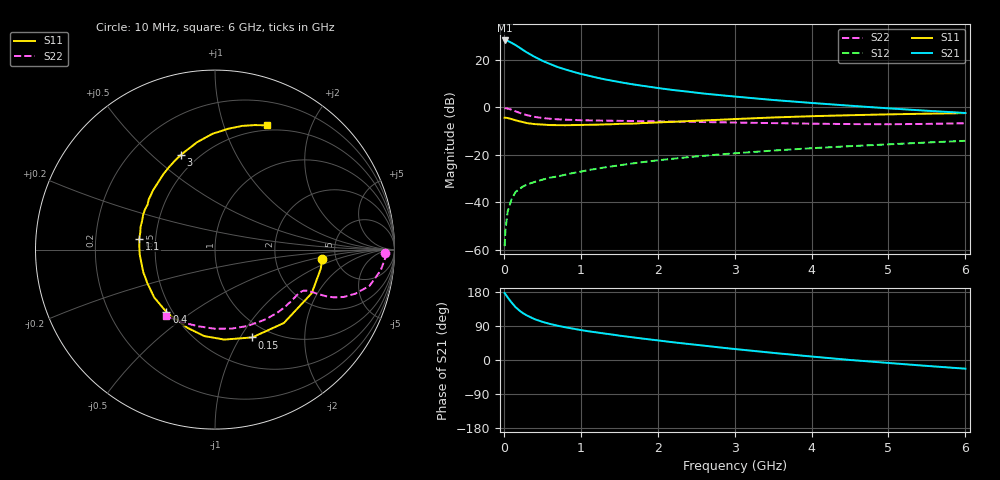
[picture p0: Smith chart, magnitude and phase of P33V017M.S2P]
! SIEMENS Small Signal Semiconductors
! BFP181
! Si NPN RF Bipolar Junction Transistor in SOT143
! VCE = 3 V  IC = 17 mA
! Common Emitter S-Parameters:  March  1996
# GHz  S  MA  R  50
!  f  S11  S21  S12  S22
! GHz  MAG  ANG  MAG  ANG  MAG  ANG  MAG  ANG
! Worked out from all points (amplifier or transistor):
!   36 points, 10 MHz to 6 GHz, reference 50 ohm
!   highest |S21| = 28.0 dB at 10 MHz (marker M1)
!   |S21| within 3 dB of that: start of sweep to 203.9 MHz
!   unconditionally stable (mu >= 1): start of sweep to 11.11 MHz; 618.9 MHz to end of sweep
!   at 250 MHz: K = 0.55, MSG = 28.7 dB, |S12| = -33.4 dB
!   at 1.4 GHz: K = 1.32, MAG = 14.7 dB, |S12| = -24.9 dB
!   at 6 GHz: K = 1.07, MAG = 4.3 dB, |S12| = -14.2 dB
!   S11 on the Smith chart (normalised r, x): 10 MHz: 3.88, -0.62; 150 MHz: 0.83, -1.13; 400 MHz: 0.46, -0.40; 1.1 GHz: 0.40, +0.06; 3 GHz: 0.40, +0.63; 6 GHz: 0.44, +1.40
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0.01  0.5987 -4.9  25.19 176.8  0.0012 83.5  0.9487 -1.1
0.02  0.599 -10.2  25.14 174.1  0.0025 80.1  0.9503 -2.7
0.05  0.5911 -24.3  24.63 165.1  0.0065 83.3  0.9308 -7.1
0.1  0.5608 -46.8  22.5 151.7  0.0116 68.2  0.8843 -13.2
0.15  0.5315 -67.0  20.27 140.0  0.0163 63.6  0.8203 -17.4
0.2  0.504 -84.1  18.01 130.8  0.0191 58.5  0.7643 -20.2
0.25  0.4853 -97.2  15.86 123.4  0.0215 55.3  0.7168 -21.8
0.3  0.4619 -109.6  14.1 117.5  0.0237 54.5  0.6789 -22.7
0.4  0.4406 -127.9  11.4 107.8  0.0269 52.5  0.6254 -23.3
0.5  0.431 -141.8  9.434 100.8  0.0299 51.3  0.5917 -23.6
0.6  0.4207 -153.3  8.077 95.2  0.033 51.9  0.5704 -23.9
0.7  0.4188 -162.4  6.952 90.4  0.0351 52.7  0.5552 -24.3
0.9  0.4203 -176.4  5.547 82.7  0.0413 53.9  0.5382 -25.5
1.1  0.426 171.7  4.583 75.8  0.0478 54.4  0.5272 -27.4
1.5  0.445 154.1  3.369 64.4  0.0601 54.9  0.5154 -32.1
1.8  0.4633 142.9  2.816 56.6  0.0698 54.4  0.5076 -36.4
2.2  0.4916 129.9  2.292 46.8  0.0825 52.3  0.4982 -42.6
3  0.5619 109.6  1.67 29.0  0.1073 47.2  0.4744 -56.9
3.5  0.6069 99.4  1.415 18.8  0.1224 43.8  0.4623 -67.0
4.5  0.6768 83.9  1.072 0.1  0.1514 35.7  0.4411 -90.1
5.5  0.7287 72.2  0.84 -15.6  0.1808 28.0  0.4449 -114.3
6  0.7497 67.4  0.754 -22.9  0.1961 23.6  0.4593 -126.3
